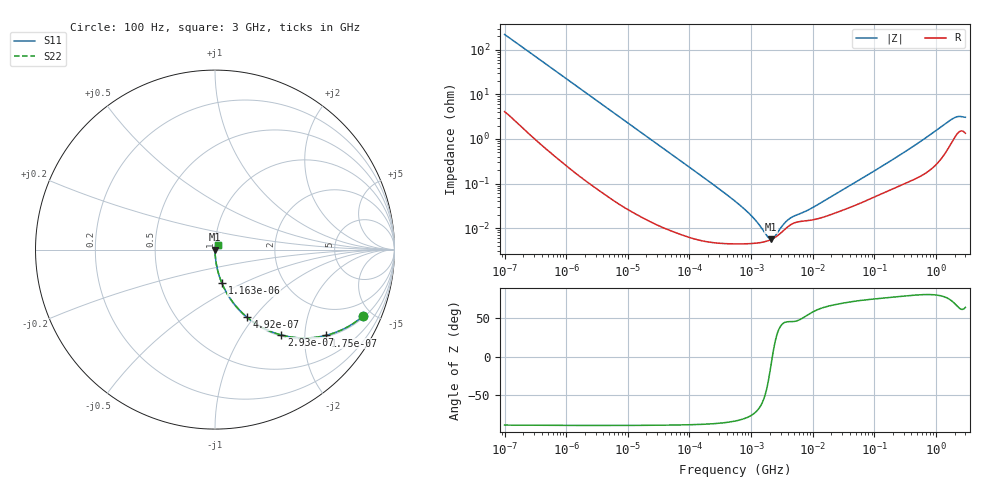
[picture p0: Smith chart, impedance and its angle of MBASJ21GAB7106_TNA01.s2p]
! MBASJ21GAB7106_TNA01  S-PARAMETER MODEL  ( Standard Model )
! Model Generated by TAIYO YUDEN Corporation (http://www.ty-top.com)
! Version 2.0
! TAIYO YUDEN Control No. 230320
! Copyright(c) 2012 TAIYO YUDEN CO.,LTD. All Rights Reserved.
! Product Description (link to TY-COMPAS)
! https://ds.yuden.co.jp/TYCOMPAS/or/detail?pn=MBASJ21GAB7106KTNA01&u=M
! Products Name : Multilayer Ceramic Capacitors
! Characteristics :
!  Capacitance : 10 [uF] , Rated Voltage : 6.3 [V] , TCC : X7R
!  Case Size : 2.0 x 1.25 / 0.079 x 0.049 [mm/inch] , Thickness : 1.25 / 0.049 [mm/inch]
!  (Conditions: Temperature = 25 [degC] , DC Bias Voltage = 0 [V])
! External Node Assignments :
!  1  o---| |---o  2
! GND o---------o GND
! Frequency Range : 100Hz  -  3GHz  [ 401 STEP ]
# MHZ S RI R 50
! Freq[MHz].  S11 Real  S11 Imag  S21 Real  S21 Imag  S12 Real  S12 Imag  S22 Real  S22 Imag
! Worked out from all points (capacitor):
!   401 points, 100 Hz to 3 GHz, reference 50 ohm
!   read as one part in series: C = 7.17 uF near 109 Hz
!   lowest |Z| = 5.66 mohm at 2.08 MHz (marker M1)
!   series resonance near 2.212 MHz, so ESL is about 720 pH
!   S11 on the Smith chart (normalised r, x): 100 Hz: 1.08, -4.42; 175 Hz: 1.04, -2.55; 293 Hz: 1.02, -1.53; 492 Hz: 1.01, -0.91; 1.163 kHz: 1.00, -0.39; 3 GHz: 1.03, +0.06
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0.0001  0.8258 -0.3701  0.1742 0.3701  0.1742 0.3701  0.8258 -0.3701
0.000175  0.6168 -0.4782  0.3832 0.4782  0.3832 0.4782  0.6168 -0.4782
0.000293  0.37 -0.4759  0.63 0.4759  0.63 0.4759  0.37 -0.4759
0.000492  0.176 -0.3746  0.824 0.3746  0.824 0.3746  0.176 -0.3746
0.000724  0.091 -0.2819  0.909 0.2819  0.909 0.2819  0.091 -0.2819
0.001163  0.0383 -0.1866  0.9617 0.1866  0.9617 0.1866  0.0383 -0.1866
0.001788  0.0171 -0.1244  0.9829 0.1244  0.9829 0.1244  0.0171 -0.1244
0.005476  0.00217 -0.0416  0.9978 0.0416  0.9978 0.0416  0.00217 -0.0416
0.031977  0.000164 -0.00721  0.9998 0.00721  0.9998 0.00721  0.000164 -0.00721
0.547723  4.45e-05 -0.000401  1 0.000401  1 0.000401  4.45e-05 -0.000401
0.918067  4.48e-05 -0.000212  1 0.000212  1 0.000212  4.48e-05 -0.000212
1.473992  4.78e-05 -8.93e-05  1 8.93e-05  1 8.93e-05  4.78e-05 -8.93e-05
1.6065  4.9e-05 -6.97e-05  1 6.97e-05  1 6.97e-05  4.9e-05 -6.97e-05
2.079876  5.5e-05 -1.32e-05  0.9999 1.32e-05  0.9999 1.32e-05  5.5e-05 -1.32e-05
2.93481  7.49e-05 5.9e-05  0.9999 -5.9e-05  0.9999 -5.9e-05  7.49e-05 5.9e-05
4.513443  0.000122 0.000124  0.9999 -0.000124  0.9999 -0.000124  0.000122 0.000124
9.794414  0.000153 0.000241  0.9998 -0.000241  0.9998 -0.000241  0.000153 0.000241
175.1444  0.000712 0.00302  0.9993 -0.00302  0.9993 -0.00302  0.000712 0.00302
513.708  0.00143 0.00797  0.9986 -0.00797  0.9986 -0.00797  0.00143 0.00797
1789.813  0.00884 0.0259  0.9912 -0.0259  0.9912 -0.0259  0.00884 0.0259
2317.205  0.0146 0.0279  0.9854 -0.0279  0.9854 -0.0279  0.0146 0.0279
3000  0.014 0.0269  0.986 -0.0269  0.986 -0.0269  0.014 0.0269
